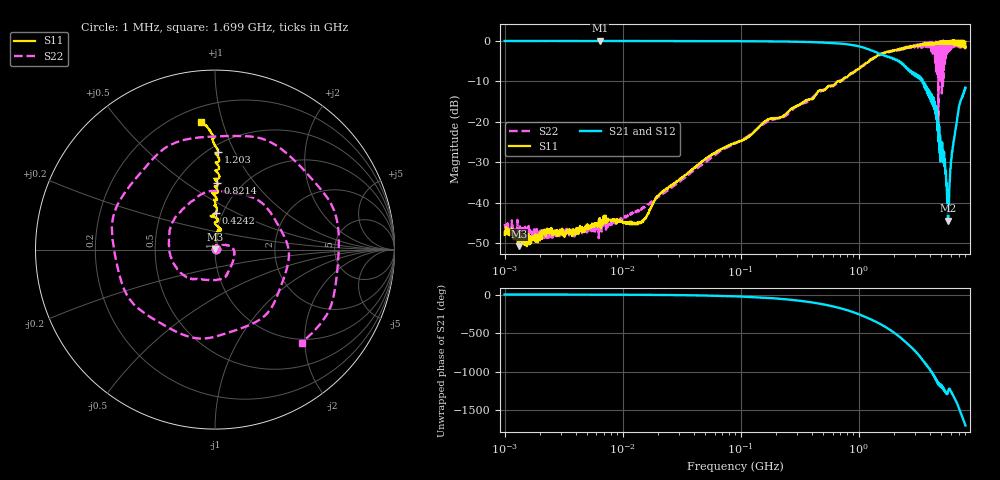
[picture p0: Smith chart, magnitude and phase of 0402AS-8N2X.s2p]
!s-Parameter Generated by FASTRON Sdn. Bhd.
!FASTRON P/N : 0402AS-8N2X
!Keysight Technologies: E5071C_MY46733604_B.14.02
!Date: Mon Dec 01 10:27:14 2025
!Version  :Rev00  Mon Dec 01 10:27:14 2025
!Data & Calibration Information:
!Freq  S11:SOLT2(ON)  S21:SOLT2(ON)  S12:SOLT2(ON)  S22:SOLT2(ON)
!PortZ  Port1:50+j0  Port2:50+j0
!When reading reference impedance value at option line is always used.
! Remarks : This data is being provided solely for informational purposes.
# Hz S dB R 50
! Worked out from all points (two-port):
!   1601 points, 1 MHz to 8 GHz, reference 50 ohm
!   highest |S21| = 0.03 dB at 6.4 MHz (marker M1); lowest = -44.5 dB at 5.724 GHz (marker M2)
!   |S21| within 3 dB of the highest: start of sweep to 1.436 GHz
!   lowest |S11| = -50.8 dB at 1.323 MHz (marker M3), VSWR 1.01, Z = 50.3 + j0.131 ohm
!   |S11| at or under -10 dB: start of sweep to 662.4 MHz; 682.8 MHz to 703.2 MHz (20.38 MHz wide, 2.94 % of centre)
!   |S22| runs from -49.0 to 0.1 dB; largest |S21 - S12| = 0.016
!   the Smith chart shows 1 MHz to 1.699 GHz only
!   S11 on the Smith chart (normalised r, x): 1 MHz: 1.01, +0.00; 424.2 MHz: 0.93, +0.40; 821.4 MHz: 0.78, +0.67; 1.203 GHz: 0.56, +0.86; 1.699 GHz: 0.29, +0.85
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1000000  -48.00 21.9  -0.05 -0.3  -0.03 -0.3  -45.30 16.1
1323440  -50.80 26.8  -0.05 -0.3  -0.02 -0.4  -47.20 4.9
4479405  -46.10 29.9  -0.05 -1.2  -0.04 -1.2  -46.60 35.7
6400096  -43.90 39.1  0.03 -1.8  0.06 -1.8  -43.90 26.0
2.00676e7  -38.30 53.3  -0.05 -5.3  -0.05 -5.2  -38.50 65.4
8.994653e7  -25.20 87.5  -0.09 -23.3  -0.09 -23.2  -25.40 31.0
4.006501e8  -14.50 94.9  -0.32 -102.0  -0.31 -102.0  -14.20 -123.0
4.241554e8  -13.70 88.7  -0.35 -108.0  -0.34 -108.0  -13.50 -129.0
8.214369e8  -8.62 88.0  -0.92 151.0  -0.91 151.0  -8.59 33.7
1.202604e9  -5.27 88.3  -2.05 54.7  -2.05 54.6  -5.17 -161.0
1.442356e9  -3.56 92.6  -3.02 -4.1  -3.01 -4.2  -3.74 76.6
1.699028e9  -2.91 96.3  -3.73 -63.9  -3.73 -63.9  -3.00 -47.0
1.7949e9  -2.75 98.0  -3.94 -86.5  -3.95 -86.6  -2.81 -93.5
2.146431e9  -2.21 103.0  -5.06 -172.0  -5.06 -172.0  -2.03 93.5
2.501569e9  -1.62 109.0  -6.50 101.0  -6.47 101.0  -1.85 -90.8
2.883048e9  -1.32 117.0  -7.84 13.9  -7.81 13.7  -1.66 86.1
3.244011e9  -1.20 124.0  -8.77 -68.2  -8.74 -68.5  -1.40 -81.4
3.588581e9  -0.74 136.0  -11.50 -156.0  -11.40 -156.0  -0.60 86.8
3.95342e9  -0.75 138.0  -13.00 115.0  -13.00 114.0  -2.06 -96.4
4.296652e9  -0.74 144.0  -15.60 45.2  -15.70 44.7  -0.32 123.0
5.724236e9  -0.24 -174.0  -44.50 -164.0  -44.50 -163.0  -1.63 -164.0
8e9  -0.28 -98.5  -11.60 105.0  -11.70 105.0  -2.05 145.0
